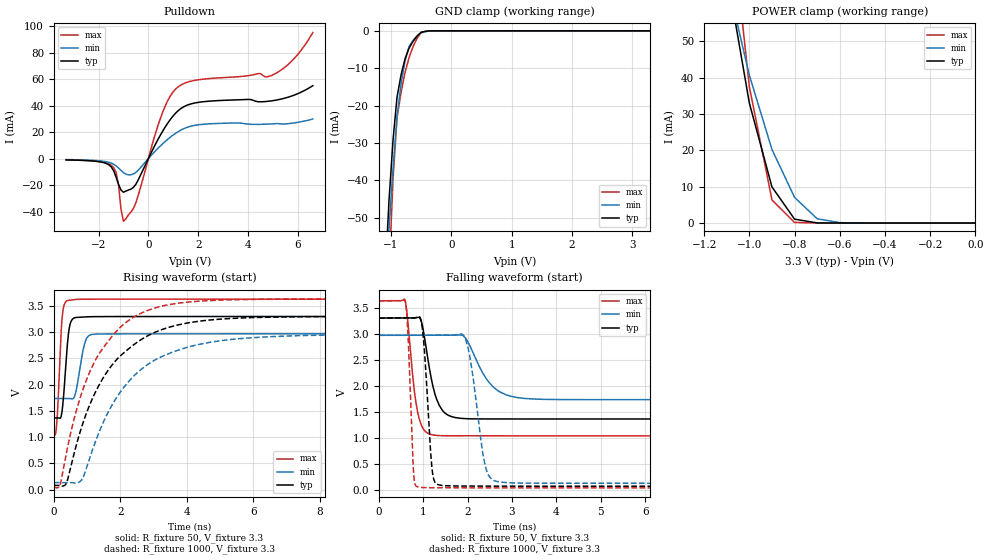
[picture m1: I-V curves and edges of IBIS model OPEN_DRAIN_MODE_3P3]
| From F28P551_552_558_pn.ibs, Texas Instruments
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|   Model Cell OPEN_DRAIN_MODE_3P3
|OPEN_DRAIN_MODE_3P3
[Model]   OPEN_DRAIN_MODE_3P3
Model_type   I/O_open_drain
Polarity   Non-Inverting
Enable   Active-Low
Vinl =  0.8
Vinh =  2
Cref =  15.0000pF
Rref =  100.0000M
Vref =  0V
Vmeas =  1.65
C_comp   1.11773p   1.013376p   1.244487p
[Model Spec]
Vinl   0.8   0.8   0.8
Vinh   2   2   2
[Temperature Range]   25   155   -40
[Voltage Range]   3.3   2.97   3.63
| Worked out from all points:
|   slope of the pulldown table from 0 to 0.495 V, typ, clamps not added: 27.3 ohm
|   GND clamp passes 1 mA (typ) near -0.54 V on its own axis
|   POWER clamp passes 1 mA (typ) near -0.79 V on its own axis
|   rising waveform, R_fixture 50, V_fixture 3.3: 20-80 % time 139ps typ, 204ps min, 112ps max; typ from 1.37 V to 3.3 V
|   rising waveform, R_fixture 1000, V_fixture 3.3: 20-80 % time 1.57ns typ, 1.73ns min, 1.34ns max; typ from 0.081 V to 3.3 V
|   falling waveform, R_fixture 50, V_fixture 3.3: 20-80 % time 266ps typ, 495ps min, 195ps max; typ from 3.3 V to 1.37 V
|   falling waveform, R_fixture 1000, V_fixture 3.3: 20-80 % time 138ps typ, 264ps min, 97ps max; typ from 3.3 V to 0.081 V
| Nom Voltages:
|   BIASFET=3.3, VDD=1.2, VDDS=3.3, VSS=0
| Min Voltages:
|   BIASFET=2.97, VDD=1.08, VDDS=2.97, VSS=0
| Max Voltages:
|   BIASFET=3.63, VDD=1.32, VDDS=3.63, VSS=0
[POWER_clamp]
|   voltage   I(typ)   I(min)   I(max)
-3.3V     1.132A     1.059A     1.769A
-1.067V   57.04mA    58.46mA    76.19mA
-1.033V   45.04mA    49.58mA    56.86mA
-1V       33.04mA    40.7mA     37.54mA
-900mV    9.95mA     20.27mA    6.36mA
-800mV    1.073mA    7.058mA    176.5uA
-700mV    35.88uA    1.186mA    3.424uA
-600mV    1.374uA    110.7uA    455.3nA
0V        338.2pA    5.96nA     285.2pA
[Pulldown]
|   voltage   I(typ)   I(min)   I(max)
-3.3V     -1.018mA   -784.1uA   -895.6uA
-1.4V     -8.945mA   -4.198mA   -6.606mA
-1.2V     -19.44mA   -7.097mA   -19.74mA
-1.1V     -23.79mA   -8.926mA   -38.1mA
-1V       -25.42mA   -10.61mA   -47.4mA
-500mV    -19.36mA   -10.45mA   -33.38mA
500mV     18.33mA    9.885mA    31.3mA
1.1V      34.47mA    19.21mA    52.67mA
2.1V      42.73mA    25.73mA    59.79mA
4.9V      43.52mA    26.17mA    62.49mA
5.8V      47.6mA     26.81mA    74.57mA
6.6V      55.08mA    29.87mA    95.23mA
[GND_clamp]
|   voltage   I(typ)   I(min)   I(max)
-3.3V     -1.198A    -966mA     -2.548A
-1.1V     -66.26mA   -70.86mA   -99.82mA
-1.033V   -45.39mA   -52.93mA   -65.1mA
-966.7mV  -29.21mA   -36.92mA   -39.58mA
-900mV    -17.69mA   -22.85mA   -23.24mA
-833.3mV  -11.79mA   -14.25mA   -16.46mA
-766.7mV  -7.428mA   -8.019mA   -11.09mA
-700mV    -4.622mA   -4.142mA   -7.129mA
-566.7mV  -1.379mA   -1.338mA   -1.958mA
-500mV    -383.7uA   -535.9uA   -452.8uA
-300mV    -821.5nA   -7.147uA   -404.1nA
3.3V      338.2pA    143.1nA    239.5pA
[Ramp]
| variable   typ   min   max
dV/dt_f  1.1674782/0.26758435n 0.74431688/0.49748067n  1.5612158/0.19548637n
dV/dt_r 16.566269m/0.16851048n 10.821448m/0.18717204n 21.089911m/0.14213015n
R_load = 50
[Rising Waveform]
R_fixture = 50
V_fixture = 3.3
V_fixture_min = 2.97
V_fixture_max = 3.63
|   time   V(typ)   V(min)   V(max)
0s        1.368V     1.738V     1.045V
85.1ps    1.368V     1.738V     1.237V
222.8ps   1.404V     1.738V     3.038V
302.4ps   1.849V     1.738V     3.503V
480.8ps   3.134V     1.739V     3.611V
650.9ps   3.28V      1.835V     3.625V
883.3ps   3.29V      2.667V     3.629V
1.085ns   3.296V     2.946V     3.63V
2.138ns   3.3V       2.969V     3.63V
500ns     3.3V       2.97V      3.63V
[Rising Waveform]
R_fixture = 1000
V_fixture = 3.3
V_fixture_min = 2.97
V_fixture_max = 3.63
|   time   V(typ)   V(min)   V(max)
0s        81.2mV     135.1mV    50.52mV
192.5ps   77.67mV    135.1mV    97.37mV
387.1ps   134.1mV    135mV      724.8mV
838.5ps   1.197V     186.7mV    1.84V
1.379ns   2.014V     1.122V     2.607V
1.98ns    2.537V     1.841V     3.081V
2.544ns   2.825V     2.247V     3.337V
3.332ns   3.068V     2.56V      3.51V
5.837ns   3.277V     2.89V      3.625V
500ns     3.3V       2.97V      3.63V
[Falling Waveform]
R_fixture = 50
V_fixture = 3.3
V_fixture_min = 2.97
V_fixture_max = 3.63
|   time   V(typ)   V(min)   V(max)
0s        3.3V       2.97V      3.63V
583ps     3.3V       2.97V      3.638V
803.8ps   3.302V     2.97V      1.863V
915.1ps   3.309V     2.97V      1.349V
1.254ns   1.867V     2.97V      1.057V
1.503ns   1.472V     2.97V      1.047V
1.948ns   1.375V     2.922V     1.047V
2.701ns   1.368V     1.897V     1.046V
4.266ns   1.368V     1.739V     1.045V
500ns     1.368V     1.738V     1.045V
[Falling Waveform]
R_fixture = 1000
V_fixture = 3.3
V_fixture_min = 2.97
V_fixture_max = 3.63
|   time   V(typ)   V(min)   V(max)
0s        3.3V       2.97V      3.63V
597.9ps   3.3V       2.97V      3.609V
783.5ps   3.301V     2.97V      294.5mV
944.1ps   3.272V     2.97V      59.09mV
1.149ns   937.5mV    2.97V      52.6mV
1.266ns   149.7mV    2.97V      52.01mV
1.948ns   84.58mV    2.907V     50.29mV
2.499ns   83.13mV    253.5mV    50.07mV
3.393ns   81.49mV    140.3mV    50.06mV
500ns     81.2mV     135.1mV    50.06mV
